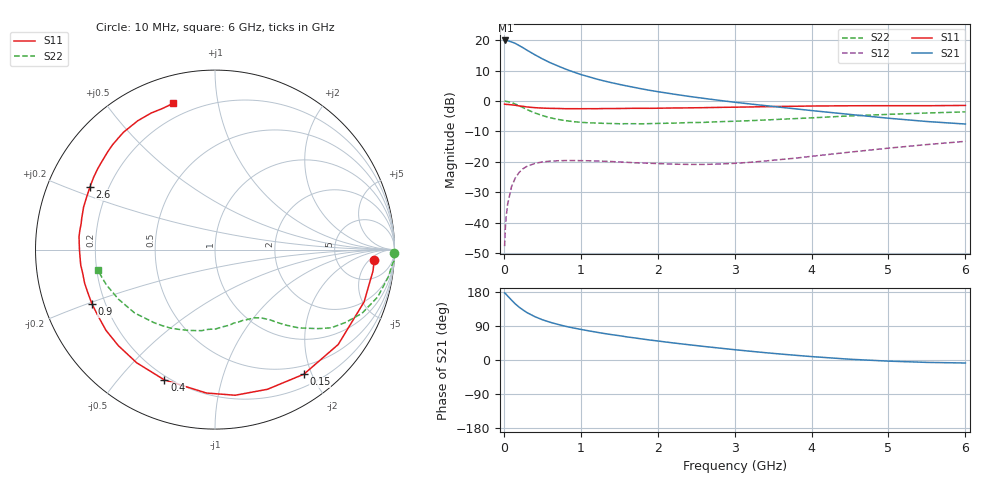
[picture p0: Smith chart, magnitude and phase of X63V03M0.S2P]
! SIEMENS Small Signal Semiconductors
! BFP193W
! Si NPN RF Bipolar Junction Transistor in SOT343
! VCE = 3 V  IC = 3 mA
! Common Emitter S-Parameters:  April 1994
# GHz  S  MA  R  50
!  f  S11  S21  S12  S22
! GHz  MAG  ANG  MAG  ANG  MAG  ANG  MAG  ANG
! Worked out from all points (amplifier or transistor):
!   40 points, 10 MHz to 6 GHz, reference 50 ohm
!   highest |S21| = 19.9 dB at 20 MHz (marker M1)
!   |S21| within 3 dB of that: start of sweep to 287.8 MHz
!   unconditionally stable (mu >= 1): 1.905 GHz to 4.591 GHz
!   at 200 MHz: K = 0.11, MSG = 20.8 dB, |S12| = -23.4 dB
!   at 1.5 GHz: K = 0.78, MSG = 12.8 dB, |S12| = -20.0 dB
!   at 6 GHz: K = 0.95, MSG = 2.8 dB, |S12| = -13.3 dB
!   S11 on the Smith chart (normalised r, x): 10 MHz: 13, -7; 150 MHz: 0.37, -1.88; 400 MHz: 0.18, -0.67; 900 MHz: 0.15, -0.21; 2.6 GHz: 0.13, +0.23; 6 GHz: 0.13, +0.75
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0.01  0.8892 -3.8  9.898 177.0  0.0041 89.6  0.9994 -1.0
0.02  0.8883 -7.8  9.938 175.5  0.0082 84.6  0.9988 -3.6
0.05  0.8804 -19.3  9.823 168.8  0.0203 80.4  0.9797 -8.6
0.1  0.8665 -37.6  9.407 158.1  0.039 69.8  0.9443 -16.2
0.15  0.8527 -54.5  8.878 147.9  0.0546 61.1  0.8928 -23.4
0.2  0.8314 -69.4  8.181 139.2  0.0673 53.8  0.8348 -29.0
0.25  0.8192 -82.1  7.538 132.0  0.0772 47.4  0.7809 -33.9
0.3  0.8005 -93.4  6.881 125.2  0.0843 42.1  0.7249 -37.4
0.4  0.7789 -111.2  5.813 114.7  0.0939 33.7  0.6398 -43.0
0.5  0.7669 -124.7  4.958 106.3  0.0997 28.0  0.5785 -46.7
0.6  0.7592 -135.2  4.294 99.7  0.1027 23.6  0.5325 -49.6
0.7  0.7558 -143.5  3.798 94.1  0.1042 20.5  0.4998 -51.7
0.9  0.7494 -156.2  3.028 84.7  0.105 15.9  0.4596 -55.9
1.1  0.7502 -165.5  2.52 77.1  0.1042 13.0  0.4387 -59.9
1.3  0.753 -173.5  2.149 70.1  0.1023 11.5  0.4299 -64.2
1.6  0.7576 177.2  1.773 61.0  0.0983 11.3  0.4242 -70.7
2.2  0.7696 162.0  1.306 45.1  0.0917 15.8  0.4331 -84.9
2.6  0.7794 153.3  1.108 35.8  0.0908 21.9  0.446 -94.8
3.2  0.7998 141.6  0.897 23.2  0.0983 32.0  0.4762 -109.4
4.5  0.8369 120.9  0.603 2.0  0.1446 42.2  0.5703 -141.8
5.5  0.8389 110.4  0.461 -6.3  0.1925 40.0  0.6364 -162.1
6  0.8476 105.9  0.419 -7.9  0.2175 37.8  0.6642 -170.2
